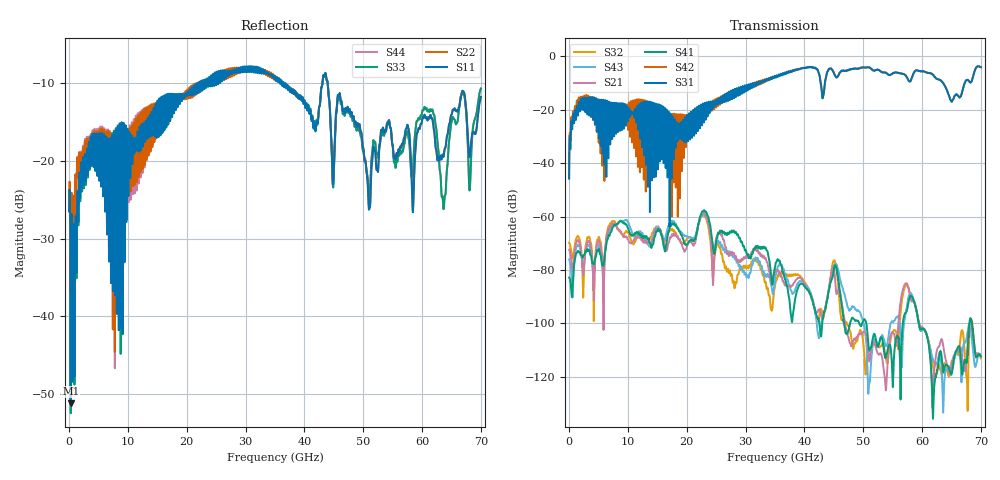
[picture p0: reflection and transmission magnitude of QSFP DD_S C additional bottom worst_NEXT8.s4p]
! AWR Design Environment (8415) Thu Dec 20 15:53:02 2018
! Document = 'CHANNEL TEST'
! nPorts: 4, nXvals: 7001
# HZ S DB R 50
!Freq DBS11 AngS11 DBS12 AngS12 DBS13 AngS13 DBS14 AngS14
!	DBS21 AngS21 DBS22 AngS22 DBS23 AngS23 DBS24 AngS24
!	DBS31 AngS31 DBS32 AngS32 DBS33 AngS33 DBS34 AngS34
!	DBS41 AngS41 DBS42 AngS42 DBS43 AngS43 DBS44 AngS44
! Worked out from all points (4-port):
!   7000 points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, 10 MHz to 70 GHz, reference 50 ohm
!   strongest paths, dB at 10 MHz, 17.51 GHz, 35.01 GHz, 52.51 GHz, 70 GHz:
!     S31: -45.8, -25.1, -7.4, -5.0, -4.0
!     S42: -45.3, -29.9, -7.6, -5.0, -4.0
!     S41: -82.8, -62.5, -78.7, -108.7, -112.2
!     S21: -72.5, -66.6, -80.8, -111.3, -112.5
!     S43: -76.1, -61.5, -84.1, -107.7, -112.6
!     S32: -69.8, -64.5, -86.0, -108.1, -113.0
!   lowest |S11| = -51.2 dB at 280 MHz (marker M1), VSWR 1.01, Z = 50.1 + j0.257 ohm
!   |S11| at or under -10 dB: start of sweep to 21.8 GHz; 36.76 GHz to 43.07 GHz (6.307 GHz wide, 15.8 % of centre); 43.96 GHz to end of sweep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
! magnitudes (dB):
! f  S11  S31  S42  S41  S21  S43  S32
! 10 MHz  -26.4  -45.8  -45.3  -82.8  -72.5  -76.1  -69.8
! 280 MHz  -51.2  -30.2  -27.5  -85.3  -74.7  -79.0  -71.7
! 2.31 GHz  -20.8  -15.5  -15.1  -75.4  -80.3  -78.1  -82.3
! 22.94 GHz  -10.5  -22.2  -20.8  -57.6  -58.4  -59.0  -59.5
! 27.08 GHz  -8.6  -16.1  -14.6  -66.3  -74.4  -73.6  -80.6
! 63.65 GHz  -19.4  -10.2  -10.2  -118.2  -109.1  -129.5  -115.5
! 70 GHz  -11.7  -4.0  -4.0  -112.2  -112.5  -112.6  -113.0
